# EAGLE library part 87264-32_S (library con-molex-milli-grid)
RECEPTACAL
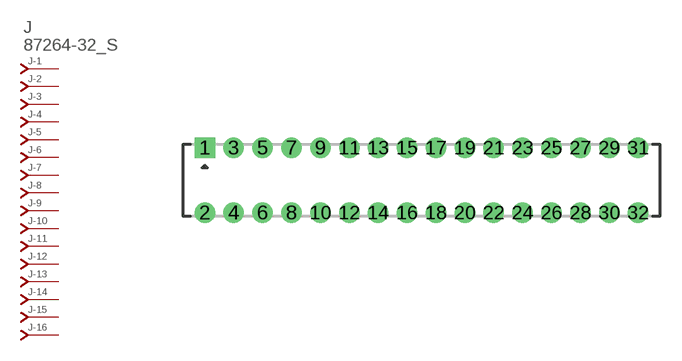
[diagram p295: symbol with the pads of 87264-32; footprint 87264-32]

Designator prefix J; gates -1=J-NV -2=J-N -3=J-N -4=J-N -5=J-N -6=J-N -7=J-N -8=J-N -9=J-N -10=J-N -11=J-N -12=J-N -13=J-N -14=J-N -15=J-N -16=J-N -17=J-N -18=J-N -19=J-N -20=J-N -21=J-N -22=J-N -23=J-N -24=J-N -25=J-N -26=J-N -27=J-N -28=J-N -29=J-N -30=J-N -31=J-N -32=J-N

## 87264-32_S  [87264-32]
1  -1:J  pas
2  -2:J  pas
3  -3:J  pas
4  -4:J  pas
5  -5:J  pas
6  -6:J  pas
7  -7:J  pas
8  -8:J  pas
9  -9:J  pas
10  -10:J  pas
11  -11:J  pas
12  -12:J  pas
13  -13:J  pas
14  -14:J  pas
15  -15:J  pas
16  -16:J  pas
17  -17:J  pas
18  -18:J  pas
19  -19:J  pas
20  -20:J  pas
21  -21:J  pas
22  -22:J  pas
23  -23:J  pas
24  -24:J  pas
25  -25:J  pas
26  -26:J  pas
27  -27:J  pas
28  -28:J  pas
29  -29:J  pas
30  -30:J  pas
31  -31:J  pas
32  -32:J  pas

## Footprint 87264-32 (pad centres in mm)
RECEPTACAL Dual Row, Side Entry
drill 0.914 square: 1 -15,2.25
drill 0.914: 2 -15,-2.25; 3 -13,2.25; 4 -13,-2.25; 5 -11,2.25; 6 -11,-2.25; 7 -9,2.25; 8 -9,-2.25; 9 -7,2.25; 10 -7,-2.25; 11 -5,2.25; 12 -5,-2.25; 13 -3,2.25; 14 -3,-2.25; 15 -1,2.25; 16 -1,-2.25; 17 1,2.25; 18 1,-2.25; 19 3,2.25; 20 3,-2.25; 21 5,2.25; 22 5,-2.25; 23 7,2.25; 24 7,-2.25; 25 9,2.25; 26 9,-2.25; 27 11,2.25; 28 11,-2.25; 29 13,2.25; 30 13,-2.25; 31 15,2.25; 32 15,-2.25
